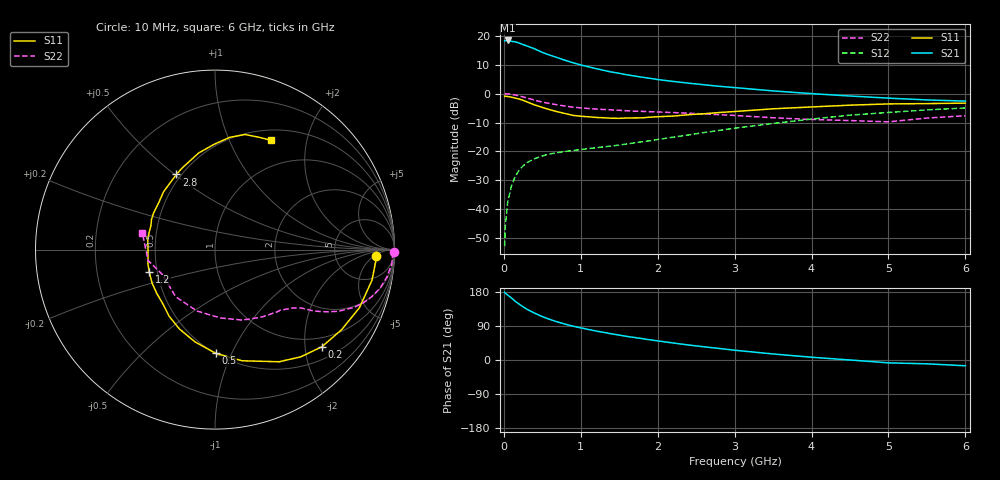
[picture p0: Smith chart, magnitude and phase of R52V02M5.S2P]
! SIEMENS Small Signal Semiconductors
! BFR183
! Si NPN RF Bipolar Junction Transistor in SOT23
! VCE = 2 V  IC = 2.5 mA
! Common Emitter S-Parameters:  May  1996
# GHz  S  MA  R  50
!  f  S11  S21  S12  S22
! GHz  MAG  ANG  MAG  ANG  MAG  ANG  MAG  ANG
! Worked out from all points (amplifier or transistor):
!   36 points, 10 MHz to 6 GHz, reference 50 ohm
!   highest |S21| = 18.4 dB at 50 MHz (marker M1)
!   |S21| within 3 dB of that: start of sweep to 407.7 MHz
!   unconditionally stable (mu >= 1): 1.304 GHz to 2.822 GHz
!   at 250 MHz: K = 0.26, MSG = 21.0 dB, |S12| = -25.0 dB
!   at 1.4 GHz: K = 1.04, MAG = 11.5 dB, |S12| = -18.1 dB
!   at 6 GHz: K = 0.91, MSG = 1.2 dB, |S12| = -5.0 dB
!   S11 on the Smith chart (normalised r, x): 10 MHz: 17, -6; 200 MHz: 0.77, -2.38; 500 MHz: 0.50, -0.87; 1.2 GHz: 0.45, -0.13; 2.8 GHz: 0.47, +0.51; 6 GHz: 0.63, +1.44
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0.01  0.8981 -2.1  8.124 178.7  0.0023 87.2  0.9951 -0.9
0.02  0.8974 -4.5  8.24 176.5  0.0052 86.1  0.9904 -1.8
0.05  0.8912 -11.0  8.296 171.5  0.0132 83.4  0.9884 -4.7
0.1  0.8675 -21.9  8.008 163.4  0.0257 77.8  0.9698 -9.1
0.15  0.8346 -32.3  7.835 154.5  0.0372 72.1  0.9433 -13.3
0.2  0.805 -42.2  7.489 147.3  0.0477 67.7  0.9103 -16.9
0.3  0.7201 -60.2  6.672 134.0  0.064 59.9  0.8402 -22.5
0.4  0.6376 -76.3  5.937 123.6  0.0749 54.1  0.7697 -26.5
0.5  0.5772 -89.7  5.156 114.4  0.0835 50.0  0.7131 -29.1
0.6  0.5258 -102.3  4.606 107.0  0.0907 47.6  0.6723 -30.8
0.7  0.4847 -114.1  4.165 100.3  0.0953 46.1  0.6373 -32.2
0.8  0.451 -124.5  3.749 94.5  0.0999 45.0  0.607 -33.2
0.9  0.4196 -133.7  3.416 89.2  0.1038 44.9  0.5827 -34.0
1.1  0.3971 -152.0  2.904 80.6  0.1118 45.6  0.5528 -36.1
1.2  0.3871 -161.0  2.701 76.4  0.1158 46.2  0.5412 -37.0
1.6  0.3791 170.9  2.113 62.2  0.1346 49.5  0.5051 -41.5
2.2  0.4085 140.0  1.624 44.9  0.1764 53.4  0.47 -50.8
2.8  0.4706 117.2  1.337 30.4  0.2308 52.8  0.4319 -63.8
3.5  0.5459 99.6  1.113 15.9  0.3047 47.5  0.382 -85.5
4.5  0.6311 82.5  0.908 0.0  0.4242 35.6  0.342 -129.9
5.5  0.6717 68.9  0.777 -10.1  0.5222 21.6  0.3772 -170.5
6  0.6839 63.0  0.741 -15.2  0.5645 12.7  0.4145 167.5
